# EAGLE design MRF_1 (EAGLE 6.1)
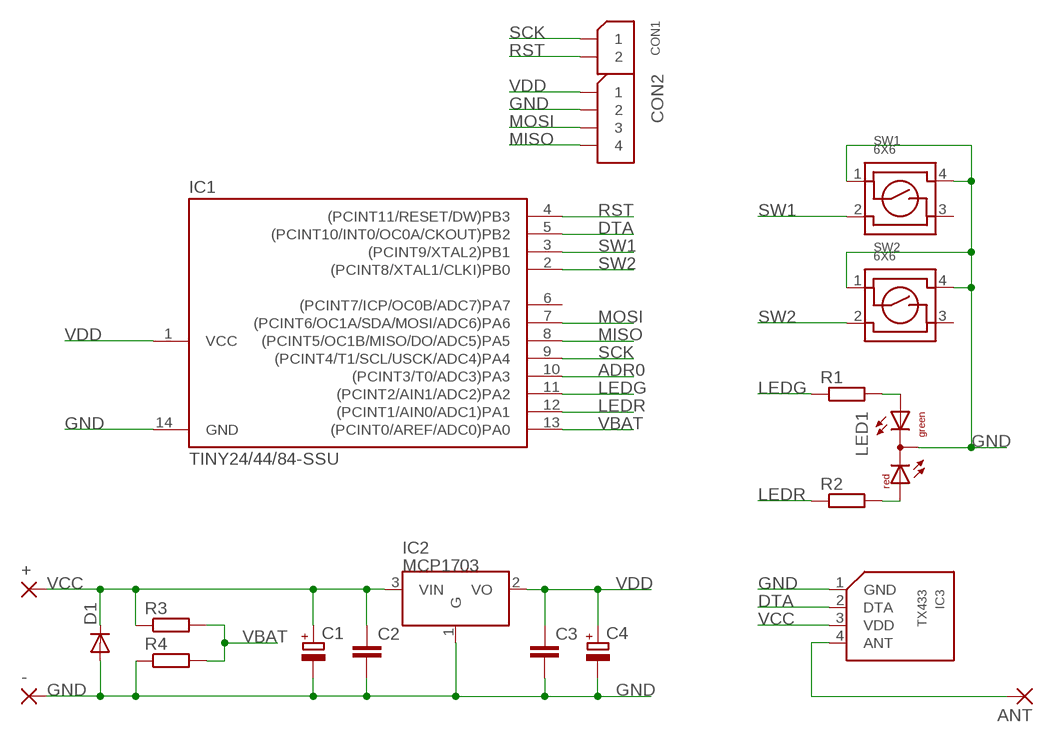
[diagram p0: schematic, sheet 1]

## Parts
+  2,15/1,0  [2,15/1,0]
-  2,15/1,0  [2,15/1,0]
ANT  2,15/1,0  [2,15/1,0]
C1  CPOL-EUSMCB  [SMC_B]
C2  C-EUC0805K  [C0805K]
C3  C-EUC0805K  [C0805K]
C4  CPOL-EUSMCB  [SMC_B]
CON1  GOLDPIN_1X2  [GOLDPIN_1X2]
CON2  GOLDPIN_1X4  [GOLDPIN_1X4]
D1  DIODE-DO214AC  [DO214AC]
IC1  TINY24/44/84-SSU  [SOIC14]
IC2  MCP1703  [SOT-23A]
IC3  TX433  [TX433]
LED1  DUOLED-RG-C  [DUOLED-C-5MM]
R1  R-EU_R0805  [R0805]
R2  R-EU_R0805  [R0805]
R3  R-EU_R0805  [R0805]
R4  R-EU_R0805  [R0805]
SW1  6X6  [6X6]
SW2  6X6  [6X6]

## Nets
ADR0: IC1.10((PCINT3/T0/ADC3)PA3)
DTA: IC1.5((PCINT10/INT0/OC0A/CKOUT)PB2) IC3.2(DTA)
GND: -.1(P) C1.- C2.2 C3.2 C4.- CON2.P$2 D1.A IC1.14(GND) IC2.1(G) IC3.1(GND) LED1.C R4.1 SW1.1 SW1.4 SW2.1 SW2.4
LEDG: IC1.11((PCINT2/AIN1/ADC2)PA2) R1.1
LEDR: IC1.12((PCINT1/AIN0/ADC1)PA1) R2.1
MISO: CON2.4 IC1.8((PCINT5/OC1B/MISO/DO/ADC5)PA5)
MOSI: CON2.P$3 IC1.7((PCINT6/OC1A/SDA/MOSI/ADC6)PA6)
N$2: LED1.AR R2.2
N$3: LED1.AX(AG) R1.2
N$6: ANT.1(P) IC3.4(ANT)
RST: CON1.2 IC1.4((PCINT11/RESET/DW)PB3)
SCK: CON1.1 IC1.9((PCINT4/T1/SCL/USCK/ADC4)PA4)
SW1: IC1.3((PCINT9/XTAL2)PB1) SW1.2
SW2: IC1.2((PCINT8/XTAL1/CLKI)PB0) SW2.2
VBAT: IC1.13((PCINT0/AREF/ADC0)PA0) R3.2 R4.2
VCC: +.1(P) C1.+ C2.1 D1.C IC2.3(VIN) IC3.3(VDD) R3.1
VDD: C3.1 C4.+ CON2.P$1 IC1.1(VCC) IC2.2(VO)
Unconnected: IC1.6((PCINT7/ICP/OC0B/ADC7)PA7) SW1.3 SW2.3

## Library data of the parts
+ - ANT = wirepad:2,15/1,0: THROUGH-HOLE PAD
C1 C4 = rcl:CPOL-EU: POLARIZED CAPACITOR, European symbol
C2 C3 = rcl:C-EU: CAPACITOR, European symbol
CON1 = DS:GOLDPIN_1X2
CON2 = DS:GOLDPIN_1X4
D1 = diode:DIODE-: DIODE
IC1 = avr-7:TINY24/44/84
IC2 = MCP1703:MCP1703
IC3 = RF:TX433
LED1 = led:DUOLED-RG-C: DUO LED 2 colors (red/green), 5 mm, round, common Cathode www.ligitek.com or other producers.
R1-R4 = rcl:R-EU_: RESISTOR, European symbol
SW1 SW2 = sw:6X6

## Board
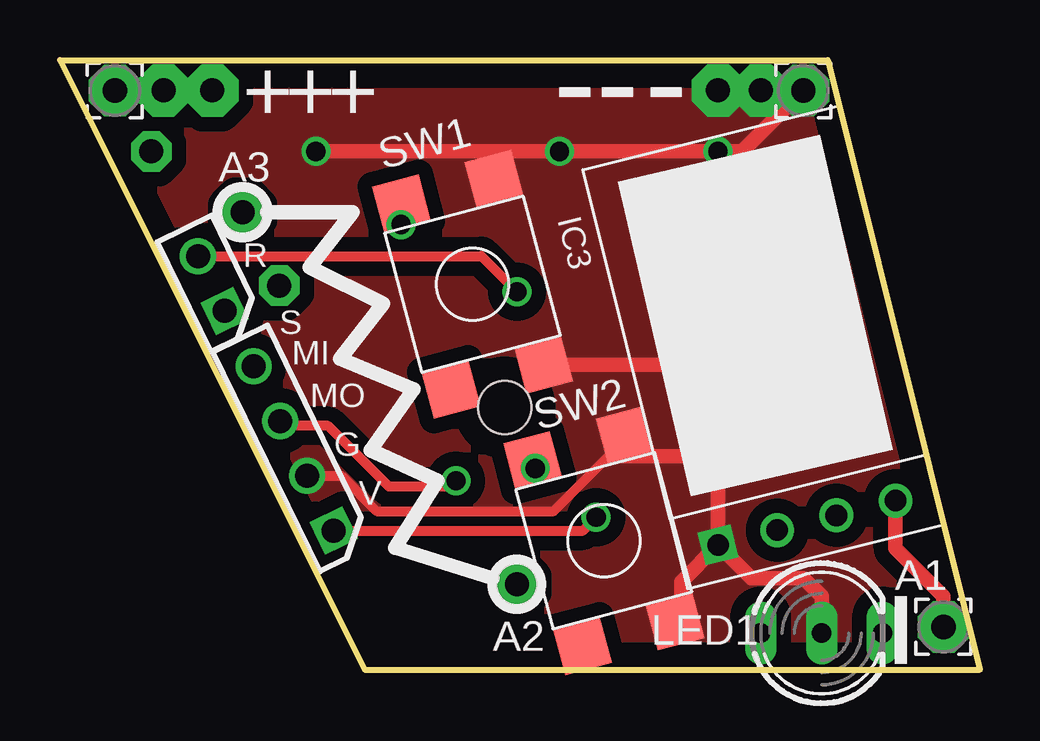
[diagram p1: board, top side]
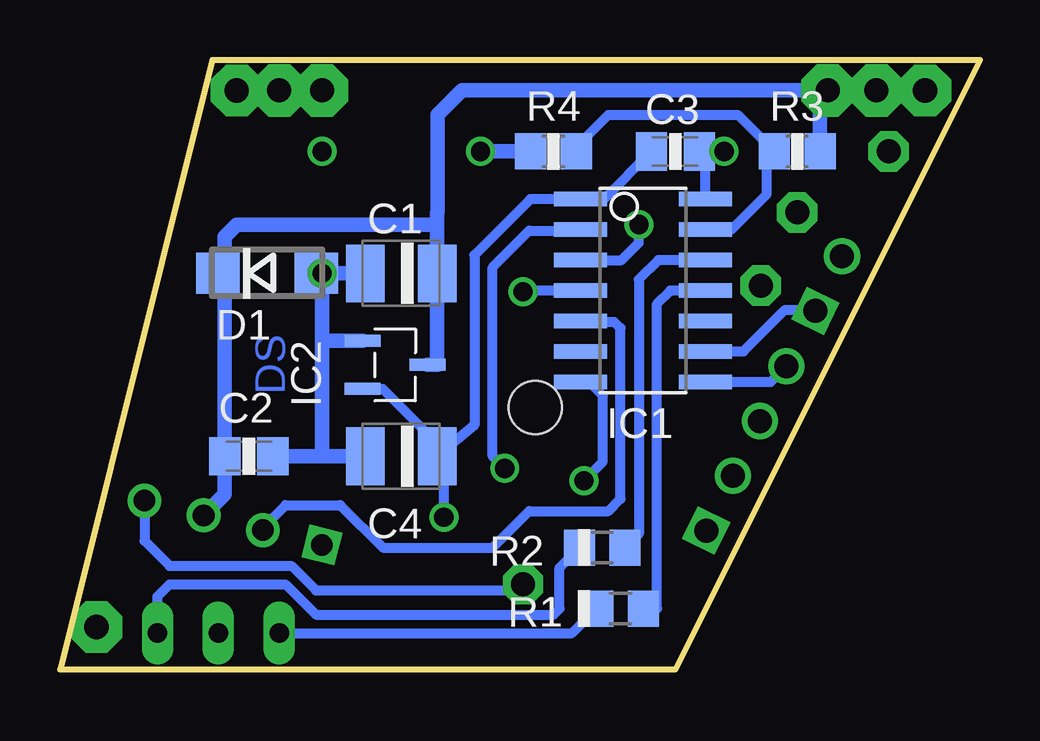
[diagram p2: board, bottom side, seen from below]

Size 38.35 x 25.4 mm. Coordinates in mm from the lower left corner, seen from the top.
Outline: 0,25.4 32,25.4 38.35,0 12.7,0 0,25.4
Copper layers (1*16): Top 0.035mm / dielectric 1.5mm / Bottom 0.035mm
Design rules: minimum track width 10mil, minimum drill 24mil, track to track 8mil, track to pad 8mil, pad to pad 8mil, via to via 8mil, smd to smd 8mil, copper to edge 40mil, drill to drill 8mil, minimum pad ring 10mil, minimum via ring 8mil, stop-mask expansion 4mil, vias tented up to drill 0mil, thermal gap 10mil
Holes 2.2 mm at 18.54,10.92

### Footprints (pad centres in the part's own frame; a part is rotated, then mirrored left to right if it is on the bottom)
2,15/1,0 = drill 1.016 pad 2.159 octagon: 1 0,0
SMC_B = smd 1.6 x 2.4: + -1.5,0; - 1.5,0
C0805K = smd 1.3 x 1.6: 1 -1,0; 2 1,0
GOLDPIN_1X2 = drill 1 square: 1 -1.27,0 | drill 1: 2 1.27,0
GOLDPIN_1X4 = drill 1: 4 3.81,0; P$2 -1.27,0; P$3 1.27,0 | drill 1 square: P$1 -3.81,0
DO214AC = smd 1.8 x 1.7: A 2.05,0; C -2.05,0
SOIC14 = smd 0.61 x 2.21: 1 -3.81,-2.603; 2 -2.54,-2.603; 3 -1.27,-2.603; 4 0,-2.603; 5 1.27,-2.603; 6 2.54,-2.603; 7 3.81,-2.603; 8 3.81,2.603; 9 2.54,2.603; 10 1.27,2.603; 11 0,2.603; 12 -1.27,2.603; 13 -2.54,2.603; 14 -3.81,2.603
SOT-23A = smd 0.5 x 1.5: 1 -1,-1.1; 2 1,-1.1; 3 0,1.6
TX433 = drill 0.9 square: 1 -3.81,-2.54 | drill 0.9: 2 -1.27,-2.54; 3 1.27,-2.54; 4 3.81,-2.54
DUOLED-C-5MM = drill 0.813 long: AR 2.54,0; AX -2.54,0; C 0,0
R0805 = smd 1.3 x 1.5: 1 -0.95,0; 2 0.95,0
6X6 = smd 2 x 2: 1 -4,2; 2 -4,-2; 3 4,-2; 4 4,2

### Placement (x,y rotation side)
+  2.29,24.13 0 top
-  30.99,24.13 0 top
ANT  36.83,1.78 0 top
C1  24.13,16.51 180 bottom
C2  30.48,8.89 0 bottom
C3  12.7,21.59 0 bottom
C4  24.13,8.89 180 bottom
CON1  6.31,16.09 116 top
CON2  9.74,9.22 116 top
D1  29.72,16.51 0 bottom
IC1  14.06,15.79 270 bottom
IC2  24.64,12.7 270 bottom
IC3  30.52,8.58 14 top
LED1  31.75,1.52 0 top
R1  14.99,2.54 180 bottom
R2  15.75,5.08 180 bottom
R3  7.62,21.59 180 bottom
R4  17.78,21.59 0 bottom
SW1  17.2,16.06 285 top
SW2  22.67,5.37 285 top

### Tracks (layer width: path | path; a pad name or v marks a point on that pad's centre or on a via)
DTA
  Bottom 0.406: IC3.2 29.9,5.91 28.96,6.86 26.67,6.86 24.89,5.08 20.32,5.08 18.8,6.6 15.49,6.6 14.99,7.11 14.99,14.22 15.24,14.48 16.61,14.48 IC1.5
GND  (via drill 0.8, 1 pad 2.18)
  Top 0.406: CON2.P$2 11.74,8.07 13.21,6.6 20.57,6.6 23.11,9.14 23.11,9.29 SW2.1
  Top 0.61: LED1.C 31.75,3.05 30.99,3.81 28.82,3.81 IC3.1 | IC3.1 27.44,8.89 | 27.44,8.89 27.44,12.7 | 27.44,12.7 v27.44,16.51 v27.43,16.51 v27.43,21.59 | SW2.1 23.57,9.45 23.11,8.89 27.44,8.89 | IC3.1 25.91,3.67 25.91,2.02 SW2.4 | SW1.4 27.44,12.7 | 18.09,20.32 SW1.1 18.09,21.53 18.03,21.59 | v10.67,21.59 18.03,21.59 | 18.03,21.59 v20.83,21.59 v27.43,21.59 | v27.43,21.59 28.45,21.59 -.1
  Bottom 0.406: IC1.14 11.45,21.34 C3.2 v10.67,21.59
  Bottom 0.61: C4.- 27.43,8.89 | 27.43,8.89 27.43,13.72 | C2.2 27.43,8.89 | IC2.1 27.42,13.7 27.43,13.72 | C1.- v27.43,16.51 | 27.43,13.72 v27.43,16.51 | D1.A v27.43,16.51 | R4.1 v20.83,21.59
  other vias: 27.43,24.13 29.21,24.13
  pour Top (isolate 0.61, no thermals): 0,25.4 32,25.4 38.35,0 12.7,0
LEDG
  Bottom 0.406: R1.1 13.46,2.54 13.46,15.24 12.91,15.79 IC1.11
LEDR
  Bottom 0.406: IC1.12 13.42,17.07 14.22,16.26 14.22,5.65 R2.1
MISO
  Bottom 0.406: IC1.8 8.72,11.99 CON2.4
MOSI  (via drill 0.8)
  Top 0.406: v16.51,7.87 16.26,7.62 13.72,7.62 11.18,10.16 9.49,10.16 CON2.P$3
  Bottom 0.406: IC1.7 16.3,11.99 15.75,11.43 15.75,8.64 v16.51,7.87
N$1  (via drill 1 pad 1.68)
  other vias: 7.62,19.05
N$2
  Bottom 0.406: LED1.AR 34.29,3.05 33.78,3.56 28.96,3.56 27.69,2.29 17.78,2.29 17.53,2.54 17.53,4.25 R2.2
N$3
  Bottom 0.406: LED1.AX 17.02,1.52 16,2.54 R1.2
N$4  (via drill 1 pad 1.68)
  other vias: 9.14,16
N$5  (via drill 1 pad 1.68)
  other vias: 19.05,3.56
N$6
  Top 0.61: ANT.1 36.83,3.05 34.83,5.05 IC3.4
  Bottom 0.406: IC3.4 34.83,5.37 33.78,4.32 28.7,4.32 27.69,3.3 19.3,3.3 19.05,3.56
N$7  (via drill 1 pad 1.68)
  other vias: 3.81,21.59
RST  (via drill 0.8)
  Top 0.406: CON1.2 17.57,17.23 v19.05,15.75
  Bottom 0.406: IC1.4 19,15.79 v19.05,15.75
SCK
  Bottom 0.406: IC1.9 9.86,13.25 8.13,14.99 6.91,14.99 CON1.1
SW1  (via drill 0.8)
  Top 0.406: v14.22,18.54 14.22,19.91 SW1.2
  Bottom 0.406: IC1.3 14.94,17.07 14.22,17.78 v14.22,18.54
SW2  (via drill 0.8)
  Top 0.406: SW2.2 v19.81,8.38
  Bottom 0.406: v19.81,8.38 20.32,8.89 20.32,16.76 18.8,18.29 16.71,18.29 IC1.2
VBAT
  Bottom 0.406: R4.2 17.02,21.59 15.49,23.11 10.09,23.11 R3.2 8.89,21.27 8.89,19.81 10.37,18.34 IC1.13
VCC  (via drill 1 pad 2.18)
  Bottom 0.61: 22.63,18.54 C1.+ 22.63,12.72 22.61,12.7 IC2.3 | 22.63,18.54 22.63,19.03 22.61,19.05 22.61,23.11 21.59,24.13 6.6,24.13 | 31.5,16.51 31.5,8.91 C2.1 31.48,7.31 IC3.3 | +.1 v4.32,24.13 v6.35,24.13 6.6,24.13 | R3.1 6.67,24.06 6.6,24.13 | D1.C 31.5,16.51 | 31.5,16.51 31.5,18.03 30.99,18.54 22.63,18.54
VDD  (via drill 0.8)
  Top 0.406: CON2.P$1 21.79,5.79 v22.35,6.35
  Bottom 0.406: v22.35,6.35 22.35,8.61 C4.+ | C4.+ 21.08,10.18 21.08,17.27 18.75,19.61 IC1.1 15.69,19.61 C3.1 | C4.+ 22.63,9.42 24.89,11.68 25.72,11.68 IC2.2

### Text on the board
Bottom: DS
tPlace: + | + | + | - | - | - | SW1 | A3 | R | S | MI | SW2 | MO | G | V | A1 | A2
